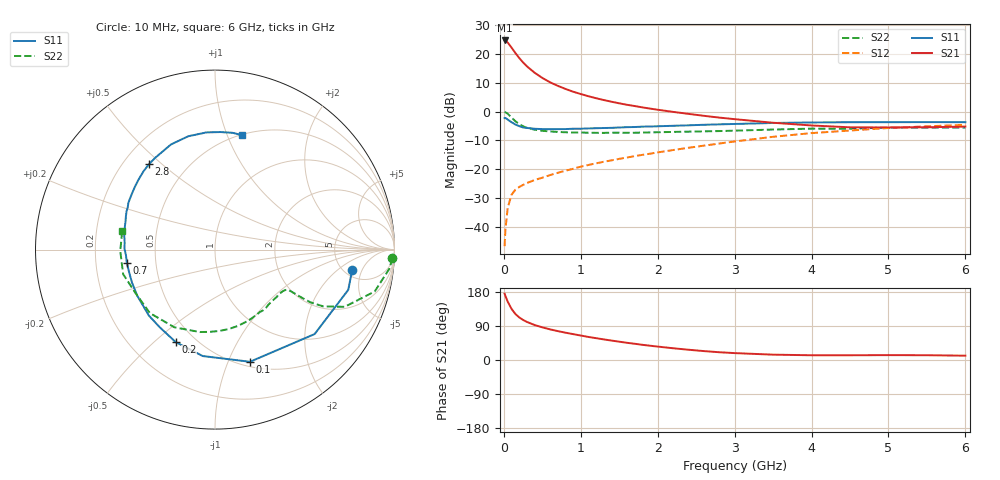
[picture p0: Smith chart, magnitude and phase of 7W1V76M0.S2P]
! Infineon Technologies  Discrete & RF Semiconductors
! BFS17W
! Si NPN RF Bipolar Junction Transistor in SOT323
! VCE = 1.75 V  IC = 6 mA
! Common Emitter S-Parameters:  August  1999
# GHz  S  MA  R  50
!  f  S11  S21  S12  S22
! GHz  MAG  ANG  MAG  ANG  MAG  ANG  MAG  ANG
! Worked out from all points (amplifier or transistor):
!   36 points, 10 MHz to 6 GHz, reference 50 ohm
!   highest |S21| = 24.7 dB at 10 MHz (marker M1)
!   |S21| within 3 dB of that: start of sweep to 114 MHz
!   unconditionally stable (mu >= 1): 481.6 MHz to 3.475 GHz; 3.529 GHz to end of sweep
!   at 250 MHz: K = 0.66, MSG = 21.3 dB, |S12| = -25.5 dB
!   at 1.4 GHz: K = 1.28, MAG = 7.0 dB, |S12| = -16.9 dB
!   at 6 GHz: K = 1.10, MAG = -2.2 dB, |S12| = -4.6 dB
!   S11 on the Smith chart (normalised r, x): 10 MHz: 5.94, -3.29; 100 MHz: 0.55, -1.20; 200 MHz: 0.39, -0.59; 700 MHz: 0.34, -0.07; 2.8 GHz: 0.30, +0.45; 6 GHz: 0.51, +1.13
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0.01  0.7728 -8.3  17.24 175.1  0.0046 83.7  0.9898 -2.8
0.02  0.7756 -16.8  17.05 169.2  0.0088 83.8  0.977 -6.3
0.05  0.7277 -40.3  15.87 154.1  0.0213 71.3  0.9198 -14.7
0.1  0.6546 -72.7  12.97 134.9  0.036 58.6  0.7897 -23.8
0.15  0.597 -96.6  10.43 121.4  0.044 50.4  0.6802 -27.7
0.2  0.56 -113.0  8.544 112.4  0.0491 49.4  0.6084 -28.9
0.25  0.5309 -125.5  7.153 105.7  0.0533 46.8  0.5573 -29.0
0.3  0.5205 -135.0  6.122 100.5  0.0575 47.3  0.5256 -28.9
0.4  0.5038 -149.3  4.74 92.3  0.0648 48.8  0.4851 -28.8
0.5  0.4976 -158.5  3.851 86.2  0.0712 51.1  0.4647 -28.8
0.6  0.4949 -165.7  3.238 80.9  0.0789 53.0  0.4526 -29.8
0.7  0.4966 -171.5  2.812 76.3  0.0865 54.6  0.4437 -31.4
0.9  0.5047 179.3  2.221 68.3  0.1017 57.3  0.4329 -35.2
1.1  0.5111 171.5  1.85 60.8  0.1184 58.9  0.43 -40.1
1.3  0.5193 164.9  1.589 54.3  0.1348 59.7  0.4273 -45.7
1.6  0.5372 156.5  1.316 45.4  0.1595 60.9  0.4285 -54.3
2.2  0.5676 141.8  0.99 31.0  0.215 61.6  0.4441 -73.7
2.8  0.6013 127.7  0.788 20.5  0.279 59.8  0.4594 -93.9
3.5  0.6352 112.7  0.641 14.1  0.3654 54.5  0.4884 -117.5
4.5  0.6547 94.2  0.534 12.5  0.4696 42.6  0.5048 -151.4
5.5  0.658 81.4  0.535 12.6  0.5558 30.7  0.5278 -179.1
6  0.6552 76.5  0.551 11.4  0.5897 25.0  0.5274 168.6
